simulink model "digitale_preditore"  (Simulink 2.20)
settings: Solver=VariableStepDiscrete  StartTime=0.0  StopTime=10.0  RelTol=1e-3  AbsTol=1e-6
libraries: Puma x2

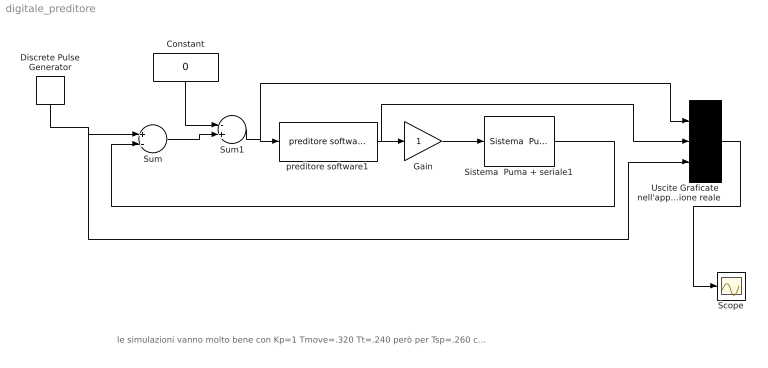
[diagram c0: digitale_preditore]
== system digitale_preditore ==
  note: le simulazioni vanno molto bene con Kp=1 Tmove=.320 Tt=.240 però per Tsp=.260 c'è un punto ad alta sensibilità
  Constant : Constant  Orientation=down  Value=0
  Discrete Pulse Generator : DiscretePulseGenerator  Orientation=down  Amplitude=48  Period=100  PulseWidth=100  PhaseDelay=1  SampleTime=.1
  Gain : Gain  Gain=1
  Scope : Scope
  Sistema  Puma + seriale1 : Puma/Sistema  Puma + seriale  Ts=.260
  Sum : Sum  Inputs=+-
  Sum1 : Sum  Inputs=-+
  Uscite Graficate  nell'applicazione reale : Mux  Inputs=3
  preditore software1 : Puma/preditore software  Tsp=.250  Tt=.240  Tmove=.320
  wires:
  Sum/1 -> Sum1/2
  Constant/1 -> Sum1/1
  Sum1/1 -> Uscite Graficate  nell'applicazione reale/1, preditore software1/1
  preditore software1/1 -> Gain/1, Uscite Graficate  nell'applicazione reale/2
  Discrete Pulse Generator/1 -> Sum/1, Uscite Graficate  nell'applicazione reale/3
  Uscite Graficate  nell'applicazione reale/1 -> Scope/1
  Sistema  Puma + seriale1/1 -> Sum/2
  Gain/1 -> Sistema  Puma + seriale1/1
